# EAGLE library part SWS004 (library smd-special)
SMD Dip Switch 4 pol.
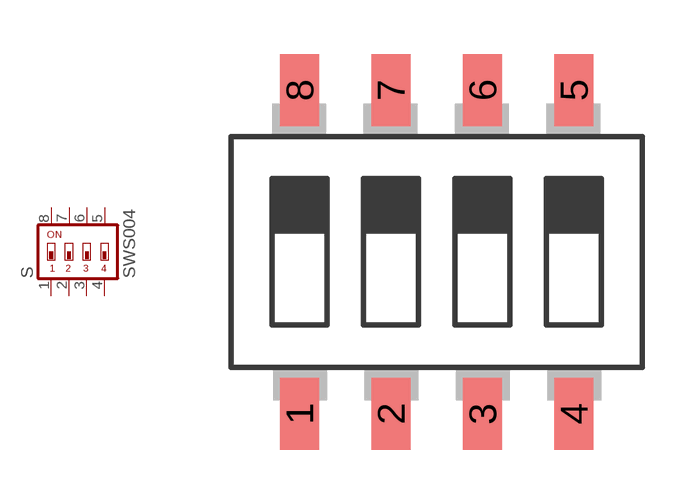
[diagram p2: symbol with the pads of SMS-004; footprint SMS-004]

Designator prefix S

## SWS004  [SMS-004]
1  1  pas
2  2  pas
3  3  pas
4  4  pas
5  5  pas
6  6  pas
7  7  pas
8  8  pas

## Footprint SMS-004 (pad centres in mm)
DIP SWITCH
smd 1.092 x 2.007: 1 -3.81,-4.496; 2 -1.27,-4.496; 3 1.27,-4.496; 4 3.81,-4.496; 5 3.81,4.496; 6 1.27,4.496; 7 -1.27,4.496; 8 -3.81,4.496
